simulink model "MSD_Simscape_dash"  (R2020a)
settings: Solver=VariableStepAuto  StartTime=0.0  StopTime=inf  MaxStep=0.1  RelTol=1e-3  EnableMultiTasking=on
libraries: fl_lib x7, nesl_utility x3

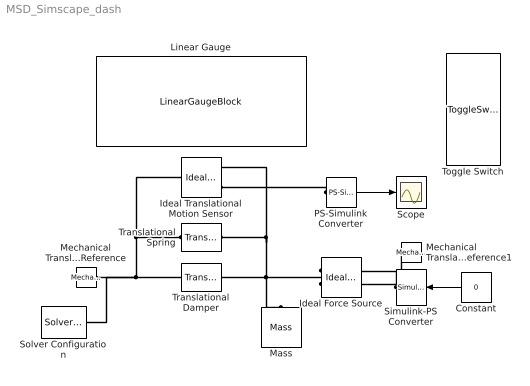
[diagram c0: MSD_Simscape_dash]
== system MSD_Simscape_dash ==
  Constant : Constant  Value=0
  Ideal Force Source : fl_lib/Mechanical/Mechanical Sources/Ideal Force Source
  Ideal Translational Motion Sensor : fl_lib/Mechanical/Mechanical Sensors/Ideal Translational Motion Sensor  offset=0 m
  Linear Gauge : LinearGaugeBlock  ScaleMin=-2  ScaleMax=2  TickInterval=1
  Mass : fl_lib/Mechanical/Translational Elements/Mass  mass=1 kg  v_specify=off  v_priority=None  v=0 m/s  v_nominal_specify=off  v_nominal_unit=m/s  v_nominal_value=1  f_specify=off  f_priority=None  f=0 N  f_nominal_specify=off  f_nominal_unit=N  f_nominal_value=1
  Mechanical Translational Reference : fl_lib/Mechanical/Translational Elements/Mechanical Translational Reference
  Mechanical Translational Reference1 : fl_lib/Mechanical/Translational Elements/Mechanical Translational Reference
  PS-Simulink Converter : nesl_utility/PS-Simulink Converter  PhysicalDomain=network_engine_domain  SubClassName=ps_output  LeftPortType=input  RightPortType=output  PseudoPeriodic=off  Frequencies=[]  Unit=m  AffineConversion=off
  Scope : Scope
  Simulink-PS Converter : nesl_utility/Simulink-PS Converter  PhysicalDomain=network_engine_domain  SubClassName=ps_input  LeftPortType=input  RightPortType=output  PseudoPeriodic=off  Frequencies=[]  NoiseDistribution=none  NoiseParameters=[]  Unit=N  AffineConversion=off  FilteringAndDerivatives=zero  SimscapeFilterOrder=1  InputFilterTimeConstant=0.001  UdotUserProvided=1
  Solver Configuration : nesl_utility/Solver Configuration  PhysicalDomain=network_engine_domain  SubClassName=solver  LeftPortType=input  RightPortType=generic  Tones=[]  Harmonics=[]  SimulateNoise=off  Profile=off  UseLocalSampling=off  EnableSwitchedLinearOptims=on  FrequencyDomain=off  UseCCode=off  RelTol=0.001  AbsTol=1e-06  MinStep=1e-09  ToWorkspace=off  RevertToSquareIcSolve=off  NumHomotopyIterations=100  PhasorMode=off  PhasorModeNumHarmonics=1  DoDC=off  ResidualTolerance=1e-09  UseLocalSolver=off  LocalSolverChoice=NE_BACKWARD_EULER_ADVANCER  LocalSolverSampleTime=0.001  DoFixedCost=off  MaxNonlinIter=3  MaxModeIter=2  LinearAlgebra=Sparse  EquationFormulation=NE_TIME_EF  DelaysMemoryBudget=1024  AutomaticFiltering=on  FilteringTimeConstant=0.001  PartitionStorageMethod=AS_NEEDED  PartitionMemoryBudget=1024  PartitionMethod=FAST
  Toggle Switch : ToggleSwitchBlock  LabelPosition=Hide
  Translational Damper : fl_lib/Mechanical/Translational Elements/Translational Damper  D=2 N/(m/s)  v_specify=off  v_priority=None  v=0 m/s  v_nominal_specify=off  v_nominal_unit=m/s  v_nominal_value=1  f_specify=off  f_priority=None  f=0 N  f_nominal_specify=off  f_nominal_unit=N  f_nominal_value=1
  Translational Spring : fl_lib/Mechanical/Translational Elements/Translational Spring  spr_rate=10 N/m  v_specify=off  v_priority=None  v=0 m/s  v_nominal_specify=off  v_nominal_unit=m/s  v_nominal_value=1  f_specify=off  f_priority=None  f=0 N  f_nominal_specify=off  f_nominal_unit=N  f_nominal_value=1  x_specify=off  x_priority=None  x=0 m  x_nominal_specify=off  x_nominal_unit=m  x_nominal_value=1
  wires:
  Constant/1 -> Simulink-PS Converter/1
  PS-Simulink Converter/1 -> Scope/1
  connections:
  Translational Spring/RConn1 -- Ideal Translational Motion Sensor/RConn1 -- Translational Damper/RConn1 -- Ideal Force Source/LConn1 -- Mass/LConn1
  Translational Spring/LConn1 -- Ideal Translational Motion Sensor/LConn1 -- Translational Damper/LConn1 -- Solver Configuration/RConn1 -- Mechanical Translational Reference/LConn1
  Mechanical Translational Reference1/LConn1 -- Ideal Force Source/RConn2
  Simulink-PS Converter/RConn1 -- Ideal Force Source/RConn1
  PS-Simulink Converter/LConn1 -- Ideal Translational Motion Sensor/RConn3
